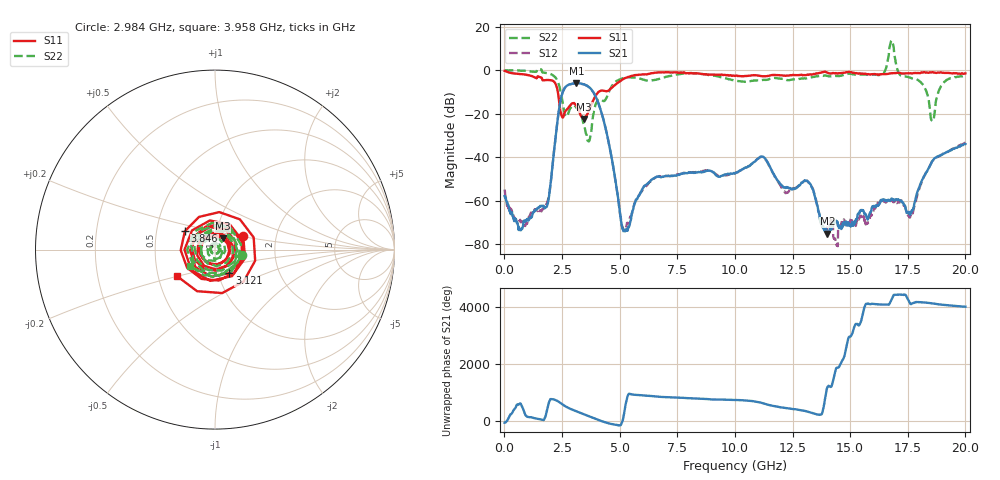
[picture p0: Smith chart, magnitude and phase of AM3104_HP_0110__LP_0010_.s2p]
!Created with skrf (http://scikit-rf.org).
# Hz S RI R 50.0
!freq ReS11 ImS11 ReS21 ImS21 ReS12 ImS12 ReS22 ImS22
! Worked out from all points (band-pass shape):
!   1601 points, 10 MHz to 20 GHz, reference 50 ohm
!   highest |S21| = -5.99 dB at 3.121 GHz (marker M1); lowest = -75.2 dB at 14.02 GHz (marker M2)
!   |S21| within 3 dB of the highest: 2.575 GHz to 3.783 GHz (1.208 GHz wide, 38 % of centre)
!   lowest |S11| = -22.4 dB at 3.458 GHz (marker M3), VSWR 1.16, Z = 53.9 + j6.85 ohm
!   |S11| at or under -10 dB: 2.319 GHz to 4.081 GHz (1.762 GHz wide, 55.1 % of centre)
!   |S22| runs from -32.7 to 13.7 dB; largest |S21 - S12| = 0.027
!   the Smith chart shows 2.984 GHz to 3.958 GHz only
!   S11 on the Smith chart (normalised r, x): 2.984 GHz: 1.36, +0.21; 3.121 GHz: 1.13, -0.31; 3.846 GHz: 0.70, +0.15; 3.958 GHz: 0.63, -0.20
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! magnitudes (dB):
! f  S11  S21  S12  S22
! 10 MHz  -0.3  -57.8  -54.9  0.0
! 697.2 MHz  -1.8  -73.5  -69.1  -0.2
! 1.822 GHz  -4.5  -63.0  -61.5  -1.2
! 2.459 GHz  -20.1  -12.8  -12.9  -10.7
! 2.984 GHz  -15.2  -6.1  -6.1  -16.3
! 3.121 GHz  -16.2  -6.0  -6.0  -17.2
! 3.346 GHz  -21.5  -6.2  -6.3  -20.7
! 3.458 GHz  -22.4  -6.5  -6.5  -25.2
! 3.846 GHz  -14.1  -9.9  -9.9  -21.1
! 3.958 GHz  -11.7  -12.1  -12.1  -15.7
! 5.182 GHz  -3.9  -73.6  -73.5  -3.5
! 6.682 GHz  -1.0  -48.9  -48.9  -4.1
! 10.01 GHz  -2.6  -47.5  -47.4  -4.8
! 11.19 GHz  -2.8  -39.8  -39.9  -4.5
! 12.19 GHz  -2.6  -54.1  -56.5  -4.3
! 13.34 GHz  -2.0  -54.0  -53.8  -3.3
! 14.02 GHz  -1.1  -75.2  -72.4  -2.6
! 16.68 GHz  -1.6  -60.0  -59.3  7.2
! 17.64 GHz  -1.4  -65.5  -67.1  -3.6
! 18.56 GHz  -0.9  -41.8  -41.8  -23.3
! 19.01 GHz  -1.2  -38.7  -38.5  -6.3
! 20 GHz  -1.5  -33.9  -33.4  -2.5
